(* Logix 5000 AddOnInstructionDefinition export V430_Monitor_Input_MXLSLC_102; software revision 33.01 *)

TYPE INPUT_MXLSLC_102 :
STRUCT
   Info : V430_InfoBits;
   Device_Status : V430_Device_Status;
   Fault_Code : DINT;
   Counters : V430_CodeReader_Counters;
   Read_Cycle_Report : V430_Read_Cycle_Report;
   Decode_Report : V430_Decode_Cycle_Report;
   Decode_Data : V430_MXLSLC_Str;
END_STRUCT
END_TYPE

TYPE OUTPUT_197 :
STRUCT
   Commands : V430_197_Commands;
END_STRUCT
END_TYPE

TYPE V430_197_Commands :
STRUCT
   Run_Mode : BOOL;
   Trigger : BOOL;
   Enable_Matchcode : BOOL;
   Reset_General_Fault : BOOL;
   Clear_NoRead_ReadCycle_Count : BOOL;
   Clear_MisMatch_ReadCycle_Count : BOOL;
   Clear_NoRead_Count : BOOL;
   Clear_Trigger_Count : BOOL;
   Clear_Matchcode_Count : BOOL;
   Clear_Mismatch_Count : BOOL;
   Output_1 : BOOL;
   Output_2 : BOOL;
   Output_3 : BOOL;
   Reserved1 : BOOL;
   Reserved2 : BOOL;
   Reserved3 : BOOL;
   Reserved4 : BOOL;
   Reserved5 : BOOL;
   Reserved6 : BOOL;
   Reserved7 : BOOL;
   Reserved8 : BOOL;
   Reserved9 : BOOL;
   Reserved10 : BOOL;
   Reserved11 : BOOL;
   Reserved12 : BOOL;
   Reserved13 : BOOL;
   Reserved14 : BOOL;
   Reserved15 : BOOL;
   Reserved16 : BOOL;
   Reserved17 : BOOL;
   Reserved18 : BOOL;
   Reserved19 : BOOL;
END_STRUCT
END_TYPE

TYPE V430_CodeReader_Counters :
STRUCT
   Noread_Read_Cycle_Counter : DINT;
   Mismatch_Per_Read_Cycle_Counter : DINT;
   No_Read_Counter : DINT;
   Trigger_Counter : DINT;
   Match_Code_Counter : DINT;
   Mismatch_Counter : DINT;
END_STRUCT
END_TYPE

TYPE V430_Decode_Cycle_Report :
STRUCT
   Decode_Location_Top : INT;
   Decode_Location_Left : INT;
   Decode_Location_Height : INT;
   Decode_Location_Width : INT;
   Code_Type : V430_Decode_Type;
   Pixels_Per_Element : REAL;
END_STRUCT
END_TYPE

TYPE V430_Decode_Type :
STRUCT
   Aztec : BOOL;
   MicroQR : BOOL;
   Postal_Code : BOOL;
   Code39 : BOOL;
   Codeabar : BOOL;
   I_2of5 : BOOL;
   UPC_EAN : BOOL;
   Code128_EAN128 : BOOL;
   Code93 : BOOL;
   PDF417 : BOOL;
   Pharmacode : BOOL;
   Data_Matrix : BOOL;
   QR_Code : BOOL;
   BC412 : BOOL;
   GS1_Databar : BOOL;
   GS1_Databar_Limited : BOOL;
   GS1_Databar_Expanded : BOOL;
   MicroPDF : BOOL;
   Composite : BOOL;
   Dot_Code : BOOL;
   Reserved_01 : BOOL;
   Reserved_02 : BOOL;
   Reserved_03 : BOOL;
   Reserved_04 : BOOL;
   Reserved_05 : BOOL;
   Reserved_06 : BOOL;
   Reserved_07 : BOOL;
   Reserved_08 : BOOL;
   Reserved_09 : BOOL;
   Reserved_10 : BOOL;
   Reserved_11 : BOOL;
   Reserved_12 : BOOL;
END_STRUCT
END_TYPE

TYPE V430_Device_Status :
STRUCT
   Run_Mode : BOOL;
   Trigger_Ack : BOOL;
   Exposure_Done : BOOL;
   Decoding : BOOL;
   Data_Is_Ready : BOOL;
   Read_Cycle_Pass : BOOL;
   Read_Cycle_Fail : BOOL;
   General_Fault : BOOL;
   New_Matchcode_Ack : BOOL;
   Matchcode_Enabled : BOOL;
   Image_Sensor_Calibrating : BOOL;
   Image_Sensor_Calibrated : BOOL;
   Training : BOOL;
   Train_Completed : BOOL;
   Optimizing : BOOL;
   Optimization_Complete : BOOL;
   Auto_Photometry_Enabled : BOOL;
   Auto_Photometry_Complete : BOOL;
   Output_1_Status : BOOL;
   Output_2_Status : BOOL;
   Output_3_Status : BOOL;
   Buffer_Overflow : BOOL;
   Reserved1 : BOOL;
   Reserved2 : BOOL;
   Reserved3 : BOOL;
   Reserved4 : BOOL; {access Read Only}
   Reserved5 : BOOL; {access Read Only}
   Reserved6 : BOOL; {access Read Only}
   Reserved7 : BOOL; {access Read Only}
   Reserved8 : BOOL; {access Read Only}
   Reserved9 : BOOL; {access Read Only}
   Reserved10 : BOOL; {access Read Only}
END_STRUCT
END_TYPE

TYPE V430_InfoBits :
STRUCT
   InfoBits : SINT;
   Reserved_01 : SINT;
   Reserved_02 : SINT;
   Reserved_03 : SINT;
END_STRUCT
END_TYPE

TYPE V430_MXLSLC_Str :   // string type
STRUCT
   LEN : DINT;
   DATA : SINT[184];
END_STRUCT
END_TYPE

TYPE V430_Read_Cycle_Report :
STRUCT
   Capture_Time : INT;
   Total_Decode_Time : INT;
   Total_ReadCycle_Time : INT;
   Reserved : INT;
END_STRUCT
END_TYPE

ADD_ON_INSTRUCTION V430_Monitor_Input_MXLSLC_102   (* revision 0.12, vendor OMRON *)
// Add On Instruction to monitor OMRON V430-F reader for good read. This AOI must use Input Assembly MXLSLC (102) and Output Assembly (197).
// Help:
// This Add-On Instruction will monitor the OMRON V430-F reader using Ethernet/IP Input Assembly MXLSLC (102) and Output Assembly (197). This AOI is used with the V430-F in Read Cycle Start/Stop or Triggered; it is not designed to be used in Presentation (Continuous) mode. This AOI is designed using the physical trigger, but will operate using the serial or  the EtherNet/IP trigger.  This AOI is also compatible with V330-F, V440-F, V460-H.
// If Start_Monitor = TRUE, the AOI logic will monitor the reader and output the barcode string on a successful barcode read.
// ----- AOI Operation, Start_Monitor = TRUE -----
// When the V430-F trigger is detected:
// Busy = TRUE, Done = FALSE, Error = FALSE, ErrorID = 0, and the Read_String will be cleared.
// If the barcode read was successful:
// Busy = FALSE, Done = TRUE, Error = FALSE, ErrorID = 0, and the Read_String contains the decoded barcode string, which can be up to 184 characters in length. ErrorMSG will be empty.
// If a no read occurs (Error):
// Busy = FALSE, Done = FALSE, Error = TRUE, ErrorID = (Positive Integer Number - see Error States below), and the Read_String will be cleared.
// These results will be retained until the next V430-F trigger is detected or the Start_Monitor = FALSE. The V430-F counters are copied into Trig_Count and Read_Count. On a good read both counters increment. On a no read, only the Trig_Count will increment.
// While waiting for the next barcode read, momentarily setting Clear_Counters = TRUE will clear the V430-F counters.
// ----- Error States -----
// ErrorID = 0, ErrorMSG =
// ErrorID = 1, ErrorMSG =  Read Cycle Failed.
// ErrorID = 2, ErrorMSG = Barcode Data cannot be stored in string data type. Null (0x00) character contained in Barcode Data.
// ErrorID = 3, ErrorMSG = Reader not in run mode.
VAR_IN_OUT
   Assembly_Input : INPUT_MXLSLC_102; {required}
   Assembly_Output : OUTPUT_197; {required}
   Barcode : V430_MXLSLC_Str; {required}
   ErrorMSG : V430_MXLSLC_Str; {required}
END_VAR
VAR_OUTPUT
   ErrorID : INT; {access Read Only, visible}
END_VAR
VAR_INPUT
   Start_Monitor : BOOL; {required}
END_VAR
VAR_OUTPUT
   Monitor_Active : BOOL; {access Read Only, visible}
   Done : BOOL; {access Read Only, visible}
   Busy : BOOL; {access Read Only, visible}
   Error : BOOL; {access Read Only, visible}
END_VAR
VAR_INPUT
   Clear_Counters : BOOL; {visible}
END_VAR
VAR_OUTPUT
   Trig_Count : DINT; {access Read Only, visible}
   Read_Count : DINT; {access Read Only, visible}
   Sequencer : ALIAS FOR State; {access None}
END_VAR
VAR
   WaitOfflineComplete : BOOL; {access None}
   WaitOfflineActive : BOOL; {access None}
   TmrOffline : TIMER := (PRE := 500); {access None}
   State : INT; {access None}
   Null_Pos : INT; {access None}
   Reset_Monitor_Tags : BOOL; {access None}
   Null_String : STRING; {access None}
   Error_Enum : V430_MXLSLC_Str[4] := ([1] := 'Read Cycle Failed.', [2] := 'Barcode data cannot be stored in string data type. Null (0x00) character contained in Barcode data.', [3] := 'Reader not in run mode.'); {access None}
END_VAR

ROUTINE Logic   (* ladder *)
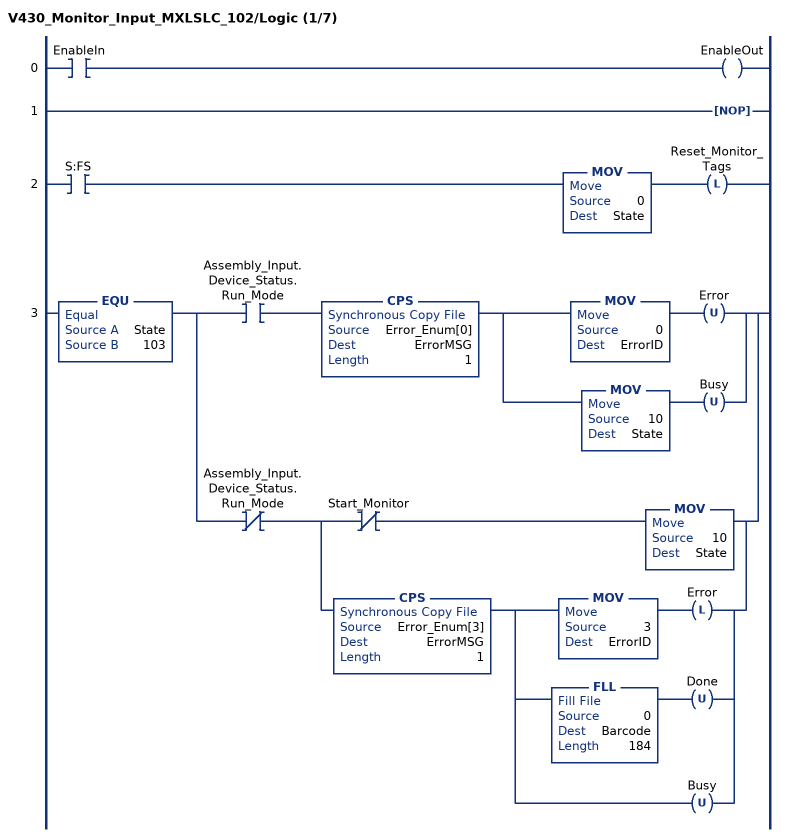
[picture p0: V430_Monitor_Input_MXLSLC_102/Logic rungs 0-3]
   0: XIC(EnableIn)OTE(EnableOut);
   1: NOP();
   2: XIC(S:FS)MOV(0,State)OTL(Reset_Monitor_Tags);
   3: EQU(State,103)[XIC(Assembly_Input.Device_Status.Run_Mode) CPS(Error_Enum[0],ErrorMSG,1) [MOV(0,ErrorID) OTU(Error) ,MOV(10,State) OTU(Busy) ] ,XIO(Assembly_Input.Device_Status.Run_Mode) [XIO(Start_Monitor) MOV(10,State) ,CPS(Error_Enum[3],ErrorMSG,1) [MOV(3,ErrorID) OTL(Error) ,FLL(0,Barcode,184) OTU(Done) ,OTU(Busy) ] ] ];
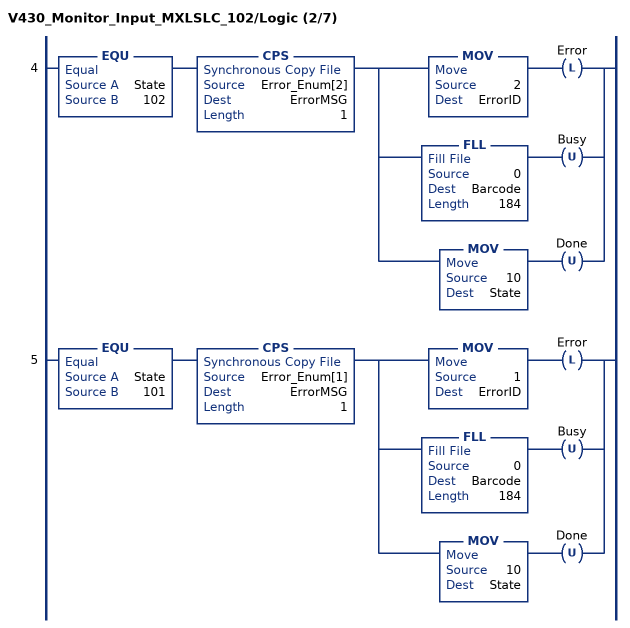
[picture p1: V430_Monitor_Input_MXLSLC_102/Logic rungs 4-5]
   4: EQU(State,102)CPS(Error_Enum[2],ErrorMSG,1)[MOV(2,ErrorID) OTL(Error) ,FLL(0,Barcode,184) OTU(Busy) ,MOV(10,State) OTU(Done) ];
   5: EQU(State,101)CPS(Error_Enum[1],ErrorMSG,1)[MOV(1,ErrorID) OTL(Error) ,FLL(0,Barcode,184) OTU(Busy) ,MOV(10,State) OTU(Done) ];
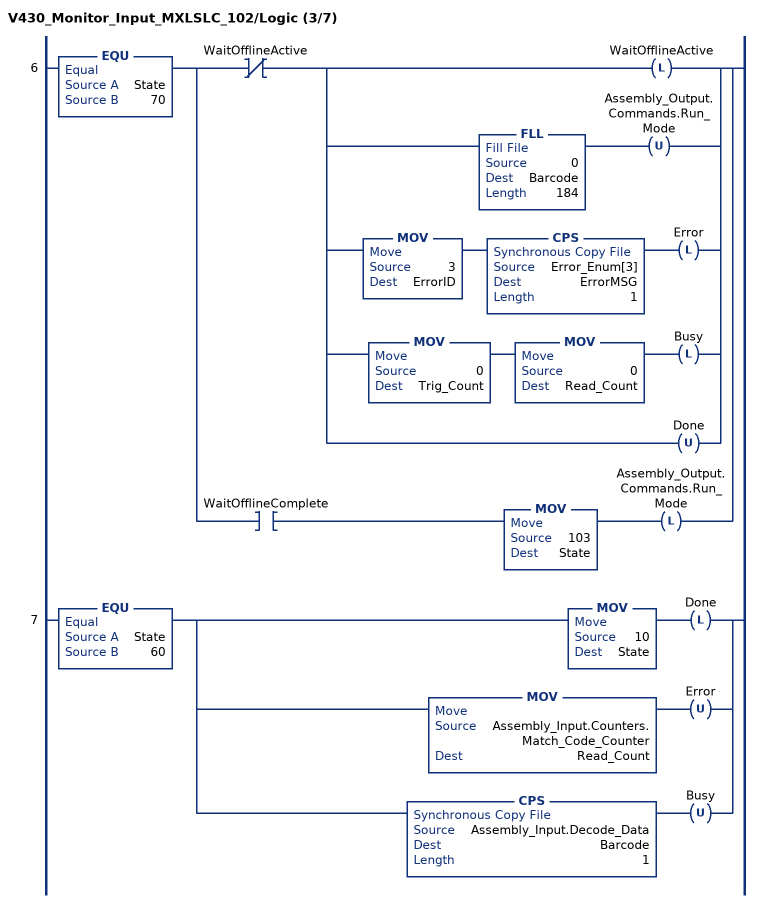
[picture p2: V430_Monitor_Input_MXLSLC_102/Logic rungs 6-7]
   6: EQU(State,70)[XIO(WaitOfflineActive) [OTL(WaitOfflineActive) ,FLL(0,Barcode,184) OTU(Assembly_Output.Commands.Run_Mode) ,MOV(3,ErrorID) CPS(Error_Enum[3],ErrorMSG,1) OTL(Error) ,MOV(0,Trig_Count) MOV(0,Read_Count) OTL(Busy) ,OTU(Done) ] ,XIC(WaitOfflineComplete) MOV(103,State) OTL(Assembly_Output.Commands.Run_Mode) ];
   7: EQU(State,60)[MOV(10,State) OTL(Done) ,MOV(Assembly_Input.Counters.Match_Code_Counter,Read_Count) OTU(Error) ,CPS(Assembly_Input.Decode_Data,Barcode,1) OTU(Busy) ];
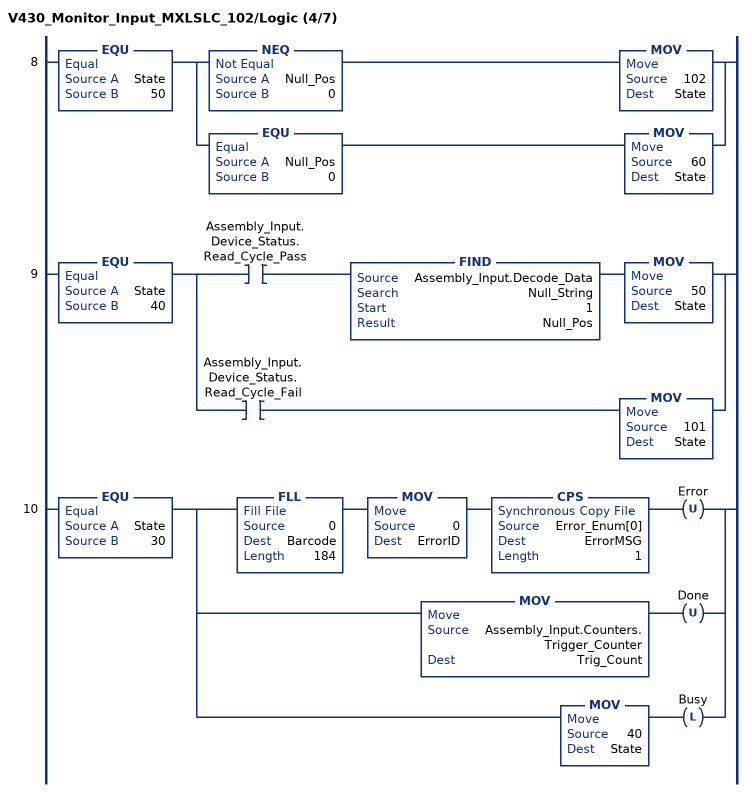
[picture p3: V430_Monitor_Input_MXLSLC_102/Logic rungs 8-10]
   8: EQU(State,50)[NEQ(Null_Pos,0) MOV(102,State) ,EQU(Null_Pos,0) MOV(60,State) ];
   9: EQU(State,40)[XIC(Assembly_Input.Device_Status.Read_Cycle_Pass) FIND(Assembly_Input.Decode_Data,Null_String,1,Null_Pos) MOV(50,State) ,XIC(Assembly_Input.Device_Status.Read_Cycle_Fail) MOV(101,State) ];
   10: EQU(State,30)[FLL(0,Barcode,184) MOV(0,ErrorID) CPS(Error_Enum[0],ErrorMSG,1) OTU(Error) ,MOV(Assembly_Input.Counters.Trigger_Counter,Trig_Count) OTU(Done) ,MOV(40,State) OTL(Busy) ];
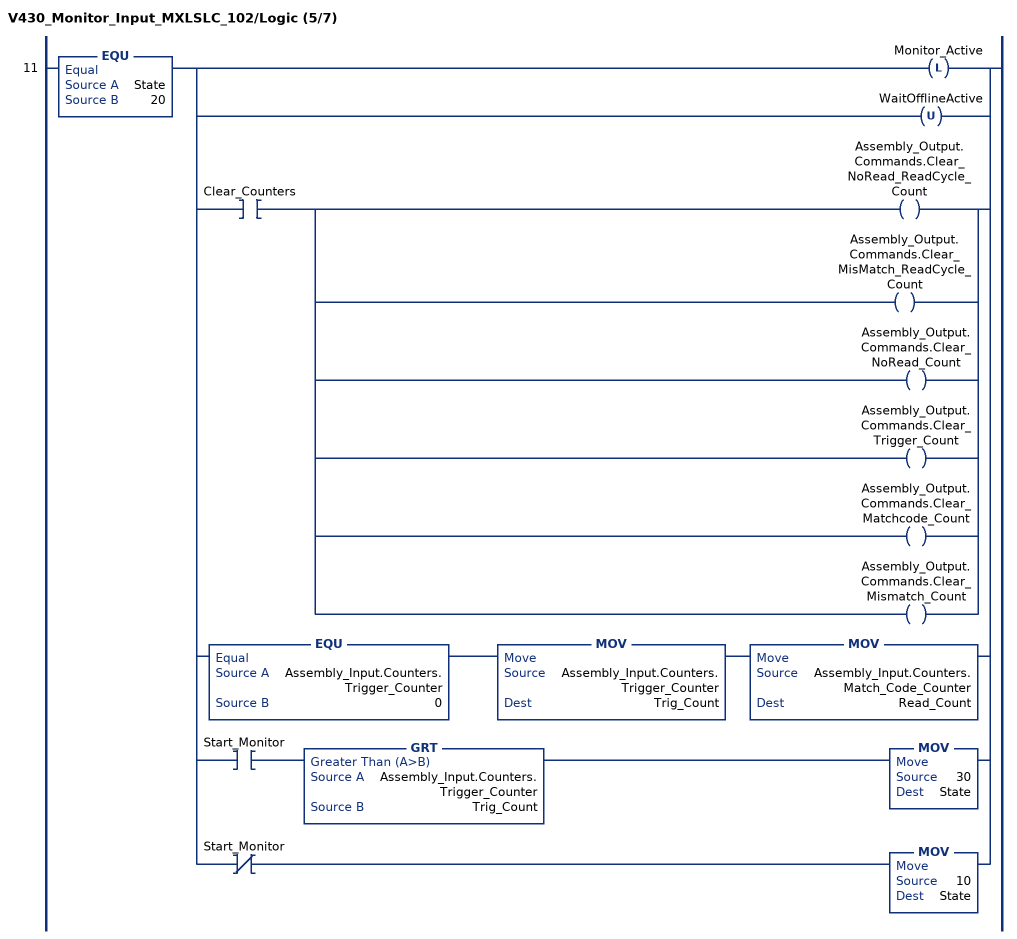
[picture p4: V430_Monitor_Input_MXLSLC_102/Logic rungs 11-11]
   11: EQU(State,20)[OTL(Monitor_Active) ,OTU(WaitOfflineActive) ,XIC(Clear_Counters) [OTE(Assembly_Output.Commands.Clear_NoRead_ReadCycle_Count) ,OTE(Assembly_Output.Commands.Clear_MisMatch_ReadCycle_Count) ,OTE(Assembly_Output.Commands.Clear_NoRead_Count) ,OTE(Assembly_Output.Commands.Clear_Trigger_Count) ,OTE(Assembly_Output.Commands.Clear_Matchcode_Count) ,OTE(Assembly_Output.Commands.Clear_Mismatch_Count) ] ,EQU(Assembly_Input.Counters.Trigger_Counter,0) MOV(Assembly_Input.Counters.Trigger_Counter,Trig_Count) MOV(Assembly_Input.Counters.Match_Code_Counter,Read_Count) ,XIC(Start_Monitor) GRT(Assembly_Input.Counters.Trigger_Counter,Trig_Count) MOV(30,State) ,XIO(Start_Monitor) MOV(10,State) ];
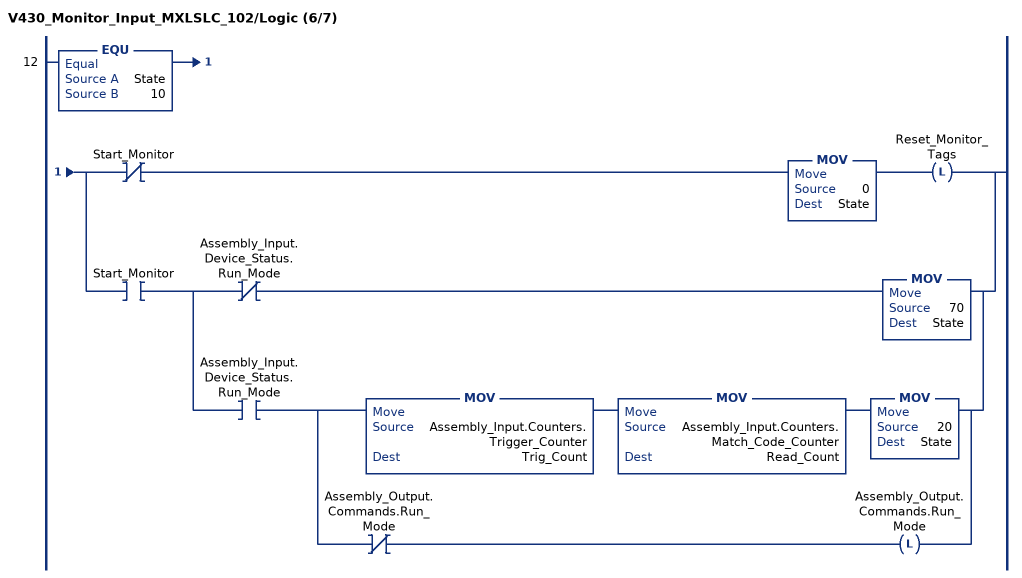
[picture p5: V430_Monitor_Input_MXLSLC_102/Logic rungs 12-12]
   12: EQU(State,10)[XIO(Start_Monitor) MOV(0,State) OTL(Reset_Monitor_Tags) ,XIC(Start_Monitor) [XIO(Assembly_Input.Device_Status.Run_Mode) MOV(70,State) ,XIC(Assembly_Input.Device_Status.Run_Mode) [MOV(Assembly_Input.Counters.Trigger_Counter,Trig_Count) MOV(Assembly_Input.Counters.Match_Code_Counter,Read_Count) MOV(20,State) ,XIO(Assembly_Output.Commands.Run_Mode) OTL(Assembly_Output.Commands.Run_Mode) ] ] ];
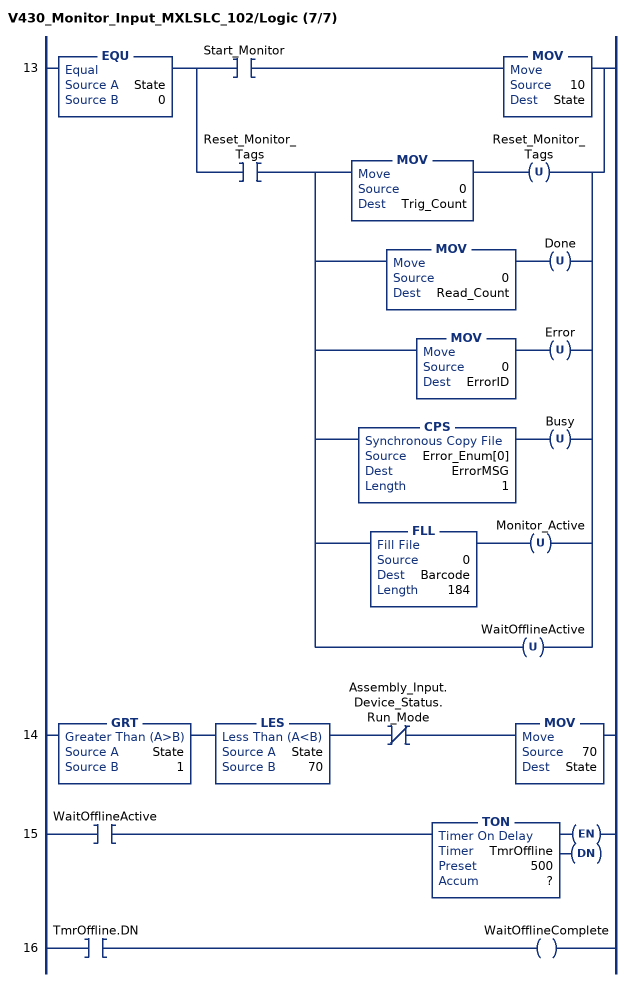
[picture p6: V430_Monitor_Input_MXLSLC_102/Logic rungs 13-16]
   13: EQU(State,0)[XIC(Start_Monitor) MOV(10,State) ,XIC(Reset_Monitor_Tags) [MOV(0,Trig_Count) OTU(Reset_Monitor_Tags) ,MOV(0,Read_Count) OTU(Done) ,MOV(0,ErrorID) OTU(Error) ,CPS(Error_Enum[0],ErrorMSG,1) OTU(Busy) ,FLL(0,Barcode,184) OTU(Monitor_Active) ,OTU(WaitOfflineActive) ] ];
   14: GRT(State,1)LES(State,70)XIO(Assembly_Input.Device_Status.Run_Mode)MOV(70,State);
   15: XIC(WaitOfflineActive)TON(TmrOffline,?,?);
   16: XIC(TmrOffline.DN)OTE(WaitOfflineComplete);
END_ROUTINE
END_ADD_ON_INSTRUCTION
